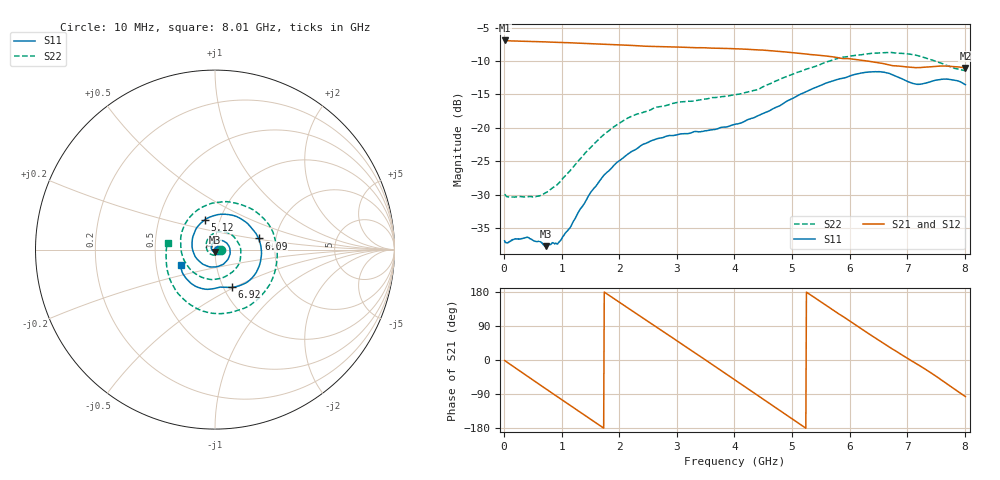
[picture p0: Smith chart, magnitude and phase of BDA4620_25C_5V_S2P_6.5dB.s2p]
!Agilent Technologies,E5071B,MY42404982,A.09.10
!Date: Wed May 06 08:59:29 2026
!Data & Calibration Information:
!Freq	S11:SOLT2(ON)	S21:SOLT2(ON)	S12:SOLT2(ON)	S22:SOLT2(ON)
# Hz S RI R 50
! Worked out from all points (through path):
!   801 points, 10 MHz to 8.01 GHz, reference 50 ohm
!   highest |S21| = -6.94 dB at 10 MHz (marker M1); lowest = -11.1 dB at 8.01 GHz (marker M2)
!   group delay of S21, straight-line fit = 283 ps
!   lowest |S11| = -37.7 dB at 720 MHz (marker M3), VSWR 1.03, Z = 50.1 - j1.29 ohm
!   |S11| at or under -10 dB: start of sweep to end of sweep
!   |S22| runs from -30.4 to -8.7 dB; largest |S21 - S12| = 0.002
!   S11 on the Smith chart (normalised r, x): 10 MHz: 1.03, -0.00; 5.12 GHz: 0.85, +0.29; 6.09 GHz: 1.62, +0.21; 6.92 GHz: 1.10, -0.49; 8.01 GHz: 0.67, -0.12
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1e7  0.0142 -0.000848  0.4498 -0.00954  0.4503 -0.00984  0.0317 -0.00246
3.4e8  0.0131 -0.00725  0.3597 -0.26  0.3602 -0.2604  0.0201 -0.0227
7.2e8  0.00155 -0.0129  0.1101 -0.4249  0.11 -0.4252  -0.0128 -0.03
9.6e8  -0.0105 -0.00931  -0.0786 -0.428  -0.0785 -0.4285  -0.0357 -0.0155
1.35e9  -0.0212 0.0142  -0.3317 -0.2713  -0.3319 -0.2717  -0.0484 0.0359
1.65e9  -0.0107 0.038  -0.4182 -0.0622  -0.4191 -0.0623  -0.0232 0.0789
1.94e9  0.0146 0.0519  -0.3893 0.1515  -0.3899 0.1518  0.0282 0.1001
2.32e9  0.0562 0.0423  -0.2038 0.3564  -0.2044 0.3567  0.1041 0.0727
2.68e9  0.0831 0.00364  0.0463 0.402  0.047 0.4024  0.1432 0.000557
2.99e9  0.0781 -0.0415  0.2476 0.3165  0.2482 0.3163  0.1338 -0.0768
3.38e9  0.0381 -0.0849  0.3883 0.0842  0.3888 0.0834  0.054 -0.1516
3.69e9  -0.0129 -0.0969  0.3709 -0.1322  0.3706 -0.1334  -0.0442 -0.1626
4.01e9  -0.0704 -0.0792  0.236 -0.3101  0.2359 -0.3108  -0.1409 -0.1066
4.52e9  -0.1278 0.0176  -0.1022 -0.3662  -0.103 -0.3667  -0.1892 0.0789
5.12e9  -0.0567 0.1667  -0.3522 -0.0773  -0.3525 -0.0765  0.000971 0.2618
5.35e9  0.0156 0.1948  -0.3454 0.0678  -0.3455 0.0682  0.1127 0.2589
5.74e9  0.1544 0.1656  -0.2123 0.2628  -0.2123 0.2635  0.2824 0.161
6.09e9  0.2425 0.0619  -0.0218 0.324  -0.0213 0.3246  0.3468 -0.0216
6.68e9  0.1817 -0.1797  0.2426 0.1679  0.2438 0.1681  0.2004 -0.3063
6.92e9  0.0959 -0.2105  0.2811 0.0615  0.2818 0.0607  0.0708 -0.3529
7.48e9  -0.0475 -0.2213  0.2176 -0.1875  0.2178 -0.1887  -0.2152 -0.2318
8.01e9  -0.1913 -0.0866  -0.0318 -0.2783  -0.0323 -0.2794  -0.2643 0.0394
